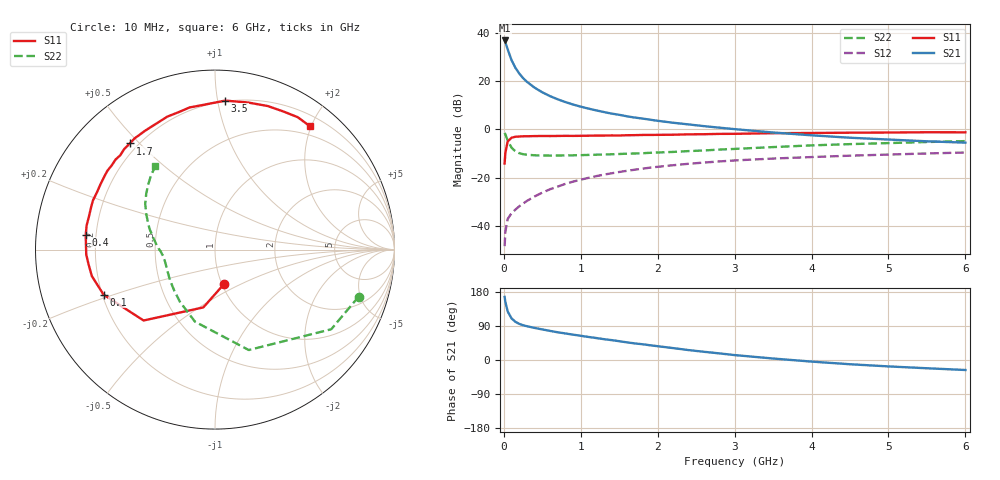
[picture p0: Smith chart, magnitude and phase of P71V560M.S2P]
! SIEMENS Small Signal Semiconductors
! BFP196
! Si NPN RF Bipolar Junction Transistor in SOT143
! VCE = 1.5 V  IC = 60 mA
! Common Emitter S-Parameters:  May  1996
# GHz  S  MA  R  50
!  f  S11  S21  S12  S22
! GHz  MAG  ANG  MAG  ANG  MAG  ANG  MAG  ANG
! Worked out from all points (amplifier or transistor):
!   36 points, 10 MHz to 6 GHz, reference 50 ohm
!   highest |S21| = 36.8 dB at 10 MHz (marker M1)
!   |S21| within 3 dB of that: start of sweep to 43.1 MHz
!   unconditionally stable (mu >= 1): 373.9 MHz to 5.106 GHz; 5.938 GHz to end of sweep
!   at 250 MHz: K = 0.90, MSG = 26.0 dB, |S12| = -30.8 dB
!   at 1.4 GHz: K = 1.10, MAG = 10.5 dB, |S12| = -18.2 dB
!   at 6 GHz: K = 1.00, MAG = 1.8 dB, |S12| = -9.6 dB
!   S11 on the Smith chart (normalised r, x): 10 MHz: 1.03, -0.41; 100 MHz: 0.20, -0.19; 400 MHz: 0.16, +0.06; 1.7 GHz: 0.17, +0.47; 3.5 GHz: 0.19, +1.05; 6 GHz: 0.36, +1.98
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0.01  0.1963 -74.4  69.35 166.4  0.0038 76.5  0.8423 -18.1
0.02  0.3285 -101.4  63.72 153.2  0.0076 68.1  0.7852 -34.4
0.05  0.5606 -135.2  45.42 128.2  0.0139 52.6  0.5904 -71.4
0.1  0.6697 -158.0  27.13 109.6  0.0183 48.7  0.4168 -105.5
0.15  0.702 -167.9  18.87 100.8  0.0217 51.1  0.3506 -123.8
0.2  0.7098 -173.7  14.38 95.4  0.0254 54.4  0.3211 -135.3
0.25  0.7179 -177.8  11.52 91.8  0.0289 56.5  0.3056 -143.7
0.3  0.7185 179.2  9.656 89.1  0.0329 59.2  0.2984 -148.9
0.4  0.7251 173.4  7.303 84.6  0.0407 62.2  0.2897 -156.7
0.5  0.7277 169.3  5.843 80.7  0.0488 63.6  0.2867 -161.8
0.6  0.7261 165.2  4.875 76.8  0.0574 64.3  0.2861 -165.1
0.7  0.7296 161.0  4.191 73.2  0.0651 64.1  0.2869 -167.7
0.9  0.731 154.3  3.266 66.9  0.0826 62.7  0.2894 -171.8
1.1  0.738 147.3  2.689 60.8  0.0989 60.8  0.2951 -174.7
1.3  0.7426 140.7  2.283 55.0  0.1153 58.2  0.3011 -177.4
1.7  0.758 128.7  1.755 43.8  0.1457 52.4  0.316 177.6
2.2  0.7738 115.3  1.369 31.4  0.1805 44.7  0.3405 171.5
2.8  0.8046 100.1  1.084 17.5  0.2162 35.6  0.3808 162.8
3.5  0.8321 86.1  0.86 3.9  0.2481 25.5  0.4288 153.1
4.5  0.8522 69.8  0.67 -11.2  0.2846 13.4  0.4938 140.9
5.5  0.8699 58.0  0.565 -21.8  0.3163 2.6  0.5461 130.8
6  0.8672 52.5  0.53 -26.4  0.3311 -3.2  0.5705 125.7
